(* Logix 5000 Controller export Example_PLC; controller Example_PLC 1769-L32E rev 19.11; software revision 19.01; part 3 of 6 *)

ADD_ON_INSTRUCTION AKD_Set_Parameter   (* revision 2.0, ExecutePrescan, ExecuteEnableInFalse *)
// Set Drive Parameter
VAR_OUTPUT
   DN : BOOL; {access Read Only, visible}   // Command Successful
   ER : BOOL; {access Read Only, visible}   // Error
END_VAR
VAR_IN_OUT
   Axis : AKD_Axis; {required}
END_VAR
VAR_INPUT
   Parameter_Number : INT; {visible}   // See help (F1) for parameter list.
   Parameter_Value : DINT; {required}   // Parameter Value
END_VAR
VAR
   Command_Timeout : TIMER := (PRE := 10000);   // Timeout Timer
   Command_Message_Type : SINT;   // Command Message Type
   Command_Axis_Number : SINT;   // Command Axis Number
   Step : SINT;
   Command_Bytes : SINT[8];
   OS_LoadStart : BOOL;
   Temp_Bytes : SINT[2];   // Temporary Bytes to Split into Command Bytes
END_VAR

ROUTINE EnableInFalse   (* ladder *)
// EnableIn_False
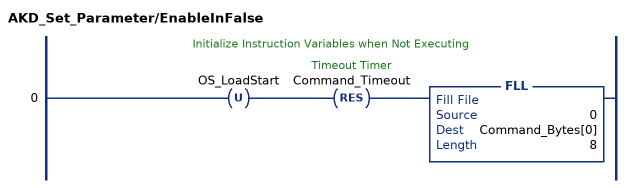
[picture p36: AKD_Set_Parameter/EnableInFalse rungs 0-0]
   // Initialize Instruction Variables when Not Executing
   0: OTU(OS_LoadStart)RES(Command_Timeout)FLL(0,Command_Bytes[0],8);
END_ROUTINE

ROUTINE Logic   (* ladder *)
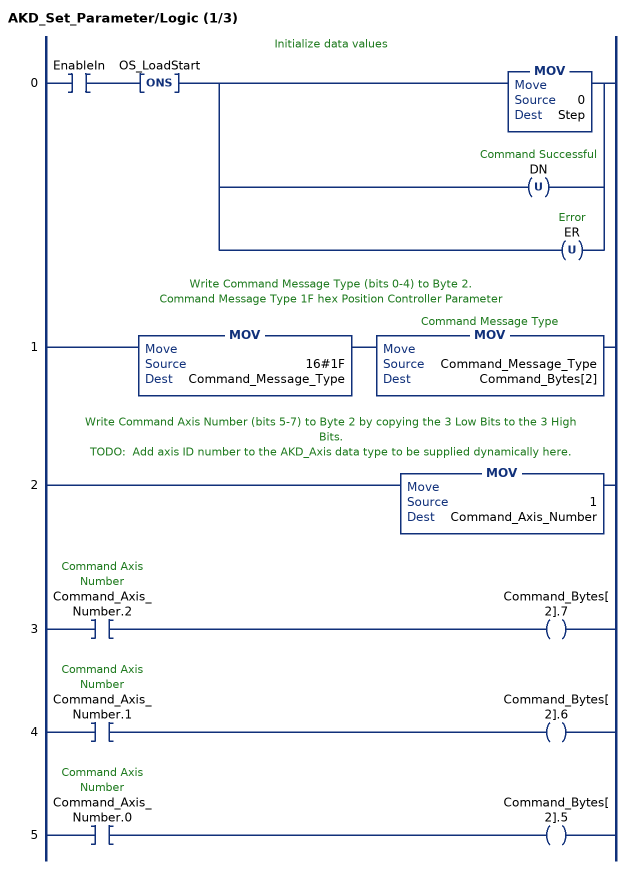
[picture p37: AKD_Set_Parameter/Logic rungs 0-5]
   // Initialize data values
   0: XIC(EnableIn)ONS(OS_LoadStart)[MOV(0,Step) ,OTU(DN) ,OTU(ER) ];
   // Write Command Message Type (bits 0-4) to Byte 2.
   // Command Message Type 1F hex Position Controller Parameter
   1: MOV(16#1F,Command_Message_Type)MOV(Command_Message_Type,Command_Bytes[2]);
   // Write Command Axis Number (bits 5-7) to Byte 2 by copying the 3 Low Bits to the 3 High Bits.
   // TODO:  Add axis ID number to the AKD_Axis data type to be supplied dynamically here.
   2: MOV(1,Command_Axis_Number);
   3: XIC(Command_Axis_Number.2)OTE(Command_Bytes[2].7);
   4: XIC(Command_Axis_Number.1)OTE(Command_Bytes[2].6);
   5: XIC(Command_Axis_Number.0)OTE(Command_Bytes[2].5);
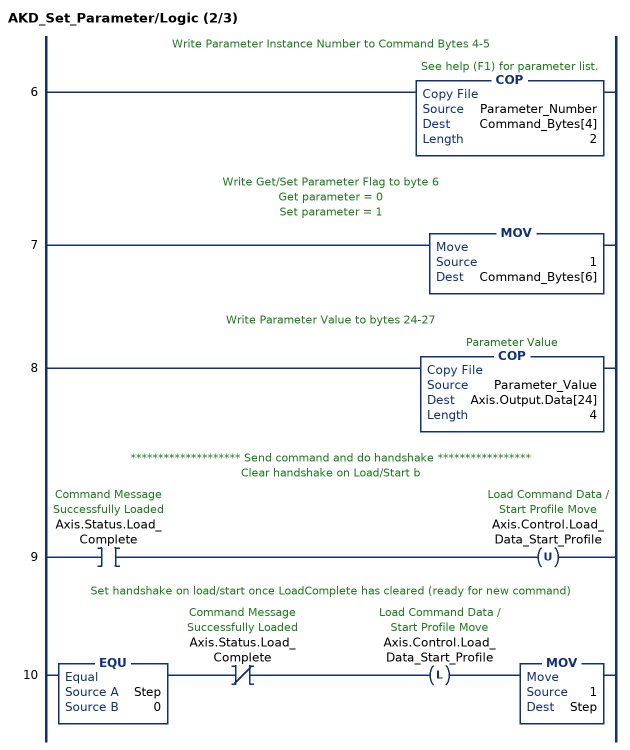
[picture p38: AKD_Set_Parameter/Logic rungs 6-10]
   // Write Parameter Instance Number to Command Bytes 4-5
   6: COP(Parameter_Number,Command_Bytes[4],2);
   // Write Get/Set Parameter Flag to byte 6
   // Get parameter = 0
   // Set parameter = 1
   7: MOV(1,Command_Bytes[6]);
   // Write Parameter Value to bytes 24-27
   8: COP(Parameter_Value,Axis.Output.Data[24],4);
   // ******************** Send command and do handshake *****************
   // Clear handshake on Load/Start b
   9: XIC(Axis.Status.Load_Complete)OTU(Axis.Control.Load_Data_Start_Profile);
   // Set handshake on load/start once LoadComplete has cleared (ready for new command)
   10: EQU(Step,0)XIO(Axis.Status.Load_Complete)OTL(Axis.Control.Load_Data_Start_Profile)MOV(1,Step);
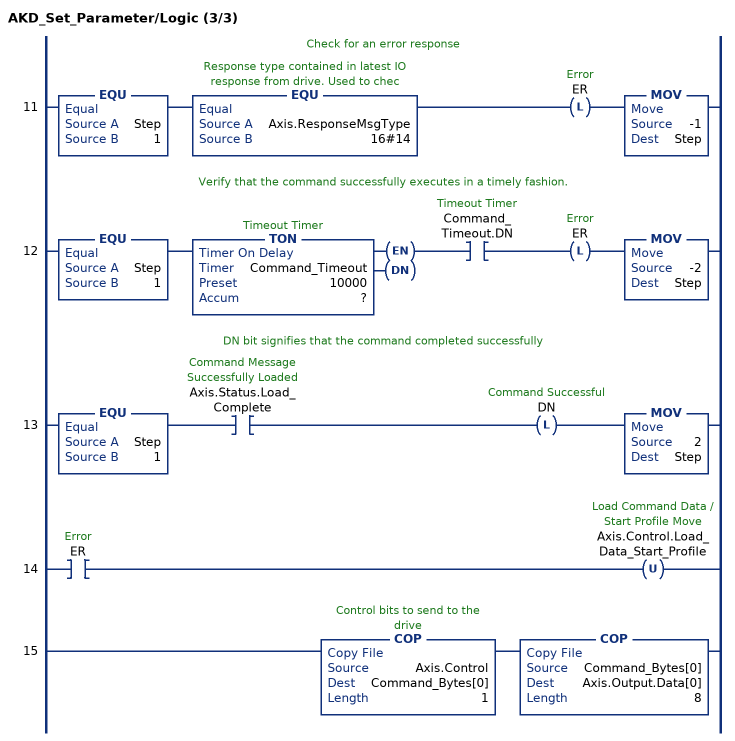
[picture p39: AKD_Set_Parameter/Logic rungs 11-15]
   // Check for an error response
   11: EQU(Step,1)EQU(Axis.ResponseMsgType,16#14)OTL(ER)MOV(-1,Step);
   // Verify that the command successfully executes in a timely fashion.
   12: EQU(Step,1)TON(Command_Timeout,?,?)XIC(Command_Timeout.DN)OTL(ER)MOV(-2,Step);
   // DN bit signifies that the command completed successfully
   13: EQU(Step,1)XIC(Axis.Status.Load_Complete)OTL(DN)MOV(2,Step);
   14: XIC(ER)OTU(Axis.Control.Load_Data_Start_Profile);
   15: COP(Axis.Control,Command_Bytes[0],1)COP(Command_Bytes[0],Axis.Output.Data[0],8);
END_ROUTINE

ROUTINE Prescan   (* ladder *)
// Prescan
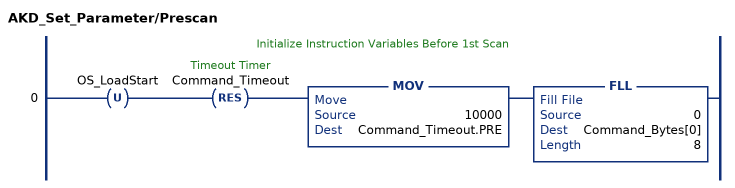
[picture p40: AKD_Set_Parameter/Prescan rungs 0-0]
   // Initialize Instruction Variables Before 1st Scan
   0: OTU(OS_LoadStart)RES(Command_Timeout)MOV(10000,Command_Timeout.PRE)FLL(0,Command_Bytes[0],8);
END_ROUTINE
END_ADD_ON_INSTRUCTION

ADD_ON_INSTRUCTION AKD_Fault_Reset_RevB   (* revision 3.0, ExecutePrescan, ExecuteEnableInFalse *)
// Drive Fault Reset
VAR_OUTPUT
   DN : BOOL; {access Read Only, visible}   // Command Successful
   ER : BOOL; {access Read Only, visible}   // Error
END_VAR
VAR_IN_OUT
   Axis : AKD_Axis; {required}
END_VAR
VAR
   Step : SINT;
   Set_Parameter : AKD_Set_Parameter := (Parameter_Number := 113);
END_VAR

ROUTINE EnableInFalse   (* ladder *)
// EnableIn_False
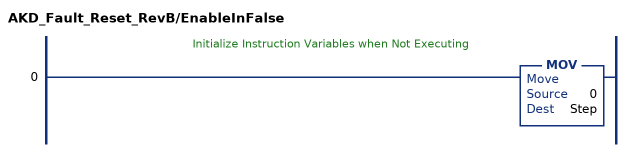
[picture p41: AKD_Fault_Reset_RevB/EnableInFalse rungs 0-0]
   // Initialize Instruction Variables when Not Executing
   0: MOV(0,Step);
END_ROUTINE

ROUTINE Logic   (* ladder *)
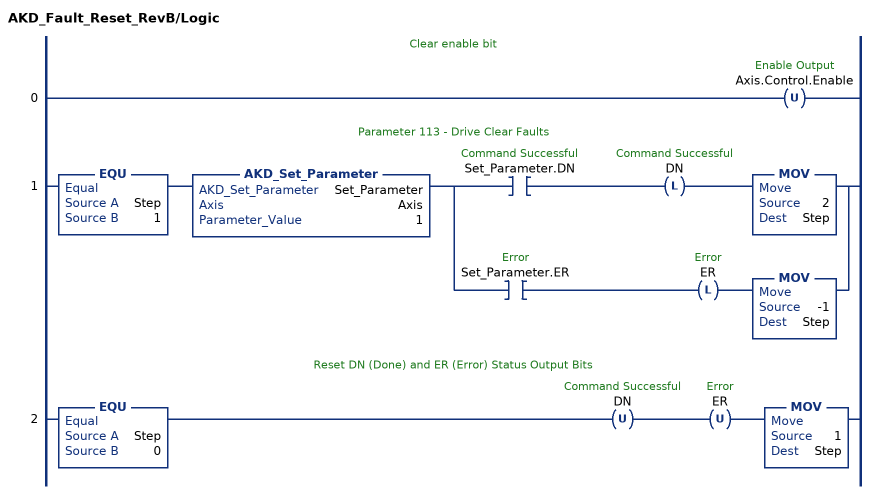
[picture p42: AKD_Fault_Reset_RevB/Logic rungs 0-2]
   // Clear enable bit
   0: OTU(Axis.Control.Enable);
   // Parameter 113 - Drive Clear Faults
   1: EQU(Step,1)AKD_Set_Parameter(Set_Parameter,Axis,1)[XIC(Set_Parameter.DN) OTL(DN) MOV(2,Step) ,XIC(Set_Parameter.ER) OTL(ER) MOV(-1,Step) ];
   // Reset DN (Done) and ER (Error) Status Output Bits
   2: EQU(Step,0)OTU(DN)OTU(ER)MOV(1,Step);
END_ROUTINE

ROUTINE Prescan   (* ladder *)
// Prescan
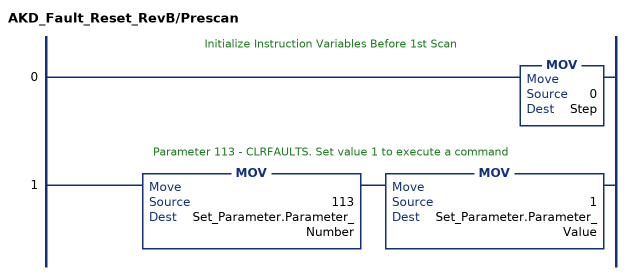
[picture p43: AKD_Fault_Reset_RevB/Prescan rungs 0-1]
   // Initialize Instruction Variables Before 1st Scan
   0: MOV(0,Step);
   // Parameter 113 - CLRFAULTS. Set value 1 to execute a command
   1: MOV(113,Set_Parameter.Parameter_Number)MOV(1,Set_Parameter.Parameter_Value);
END_ROUTINE
END_ADD_ON_INSTRUCTION

ADD_ON_INSTRUCTION AKD_Get_Attribute   (* revision 2.1, ExecutePrescan, ExecuteEnableInFalse *)
// Get Position Controller Attribute
// Revision note:
// Don't error if Command_Timeout preset is 0
VAR_OUTPUT
   DN : BOOL; {access Read Only, visible}   // Command Successful
   ER : BOOL; {access Read Only, visible}   // Error
END_VAR
VAR_IN_OUT
   Axis : AKD_Axis; {required}
END_VAR
VAR_INPUT
   Attribute_Number : INT; {visible}   // Attribute Number (see help for options)
END_VAR
VAR_OUTPUT
   Attribute_Value : DINT; {access Read Only, required}   // Attribute Value
END_VAR
VAR
   Command_Timeout : TIMER := (PRE := 100);   // Timeout Timer
   OS_LoadStart : BOOL;
   ErrorSource : SINT;
END_VAR

ROUTINE EnableInFalse   (* ladder *)
// EnableIn_False
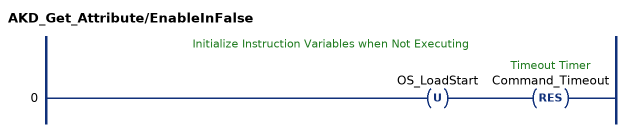
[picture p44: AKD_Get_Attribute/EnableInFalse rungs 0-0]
   // Initialize Instruction Variables when Not Executing
   0: OTU(OS_LoadStart)RES(Command_Timeout);
END_ROUTINE

ROUTINE Logic   (* ladder *)
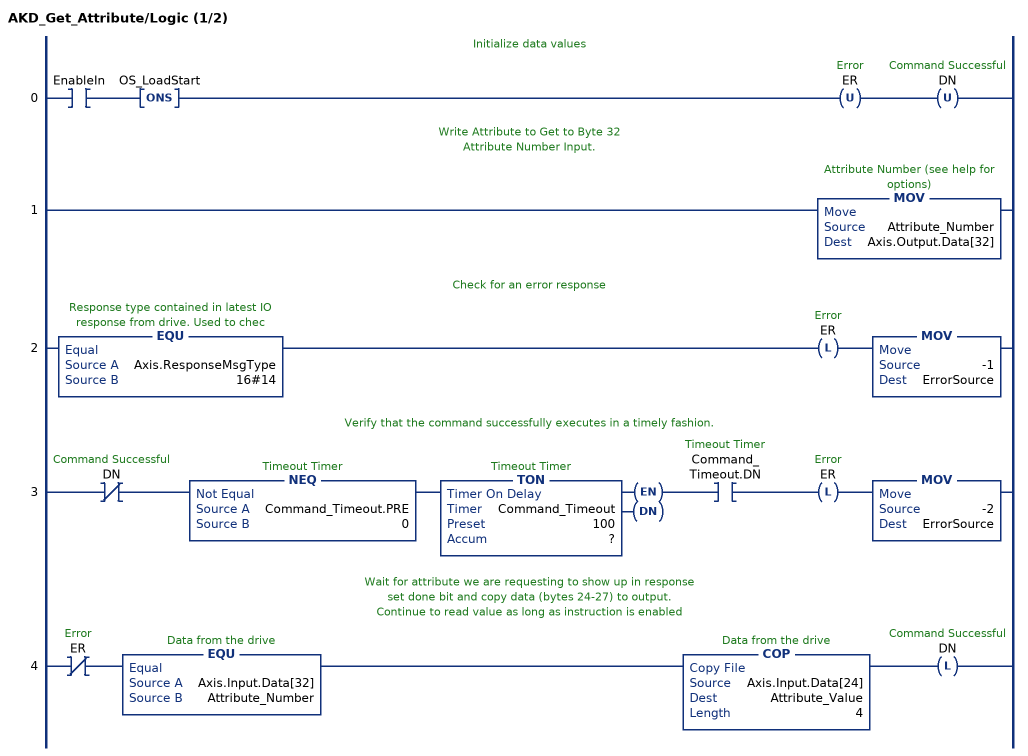
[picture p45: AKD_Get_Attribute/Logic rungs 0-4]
   // Initialize data values
   0: XIC(EnableIn)ONS(OS_LoadStart)OTU(ER)OTU(DN);
   // Write Attribute to Get to Byte 32
   // Attribute Number Input.
   1: MOV(Attribute_Number,Axis.Output.Data[32]);
   // Check for an error response
   2: EQU(Axis.ResponseMsgType,16#14)OTL(ER)MOV(-1,ErrorSource);
   // Verify that the command successfully executes in a timely fashion.
   3: XIO(DN)NEQ(Command_Timeout.PRE,0)TON(Command_Timeout,?,?)XIC(Command_Timeout.DN)OTL(ER)MOV(-2,ErrorSource);
   // Wait for attribute we are requesting to show up in response
   // set done bit and copy data (bytes 24-27) to output.
   // Continue to read value as long as instruction is enabled
   4: XIO(ER)EQU(Axis.Input.Data[32],Attribute_Number)COP(Axis.Input.Data[24],Attribute_Value,4)OTL(DN);
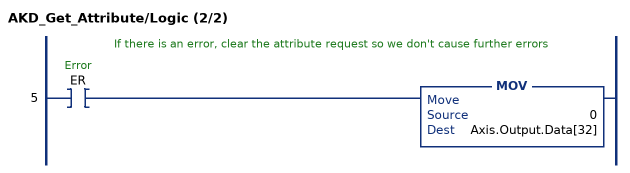
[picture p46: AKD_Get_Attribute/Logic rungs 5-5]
   // If there is an error, clear the attribute request so we don't cause further errors
   5: XIC(ER)MOV(0,Axis.Output.Data[32]);
END_ROUTINE

ROUTINE Prescan   (* ladder *)
// Prescan
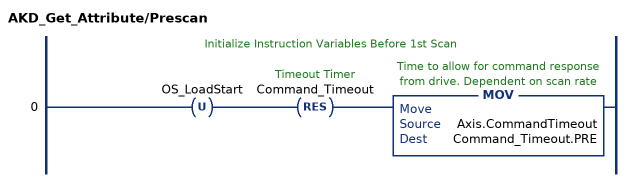
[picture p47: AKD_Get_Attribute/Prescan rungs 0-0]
   // Initialize Instruction Variables Before 1st Scan
   0: OTU(OS_LoadStart)RES(Command_Timeout)MOV(Axis.CommandTimeout,Command_Timeout.PRE);
END_ROUTINE
END_ADD_ON_INSTRUCTION

ADD_ON_INSTRUCTION AKD_Set_Attribute   (* revision 2.1, ExecutePrescan, ExecuteEnableInFalse *)
// Set Position Controller Attribute
// Revision note:
// Don't error if Command_Timeout preset is 0
VAR_OUTPUT
   DN : BOOL; {access Read Only, visible}   // Command Successful
   ER : BOOL; {access Read Only, visible}   // Error
END_VAR
VAR_IN_OUT
   Axis : AKD_Axis; {required}
END_VAR
VAR_INPUT
   Attribute_Number : INT; {visible}   // Attribute Number (see help for options)
   Attribute_Value : DINT; {required}   // Attribute Value
END_VAR
VAR
   Command_Timeout : TIMER := (PRE := 200);   // Timeout Timer
   Command_Message_Type : SINT;   // Command Message Type
   Command_Axis_Number : SINT;   // Command Axis Number
   Step : SINT;
   Command_Bytes : SINT[8];
   OS_LoadStart : BOOL;
END_VAR

ROUTINE EnableInFalse   (* ladder *)
// EnableIn_False
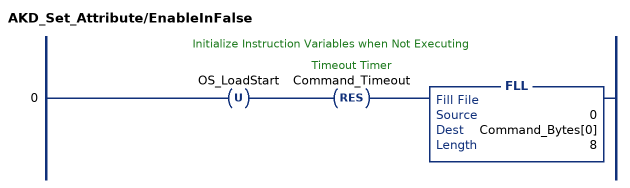
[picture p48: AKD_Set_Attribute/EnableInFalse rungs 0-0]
   // Initialize Instruction Variables when Not Executing
   0: OTU(OS_LoadStart)RES(Command_Timeout)FLL(0,Command_Bytes[0],8);
END_ROUTINE

ROUTINE Logic   (* ladder *)
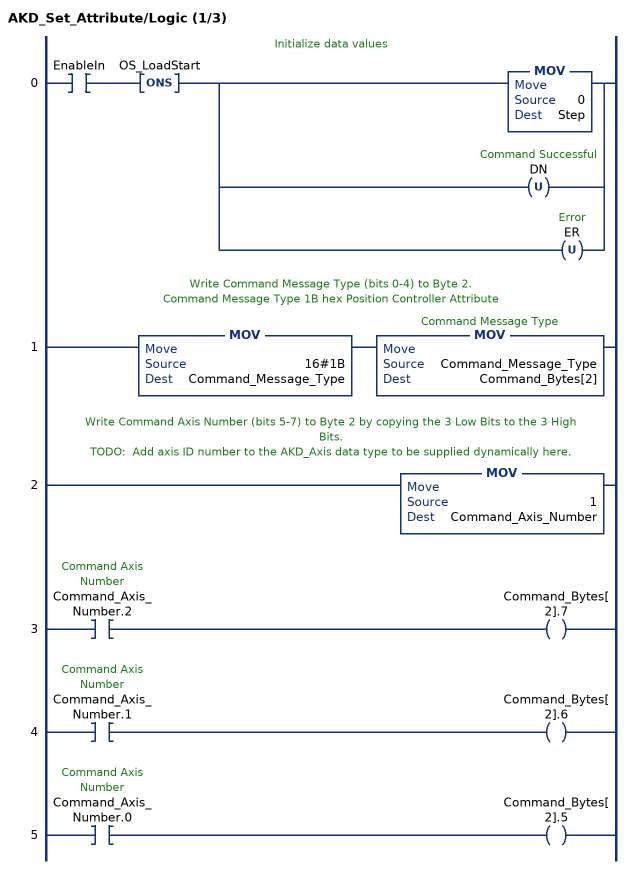
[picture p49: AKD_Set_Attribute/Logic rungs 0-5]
   // Initialize data values
   0: XIC(EnableIn)ONS(OS_LoadStart)[MOV(0,Step) ,OTU(DN) ,OTU(ER) ];
   // Write Command Message Type (bits 0-4) to Byte 2.
   // Command Message Type 1B hex Position Controller Attribute
   1: MOV(16#1B,Command_Message_Type)MOV(Command_Message_Type,Command_Bytes[2]);
   // Write Command Axis Number (bits 5-7) to Byte 2 by copying the 3 Low Bits to the 3 High Bits.
   // TODO:  Add axis ID number to the AKD_Axis data type to be supplied dynamically here.
   2: MOV(1,Command_Axis_Number);
   3: XIC(Command_Axis_Number.2)OTE(Command_Bytes[2].7);
   4: XIC(Command_Axis_Number.1)OTE(Command_Bytes[2].6);
   5: XIC(Command_Axis_Number.0)OTE(Command_Bytes[2].5);
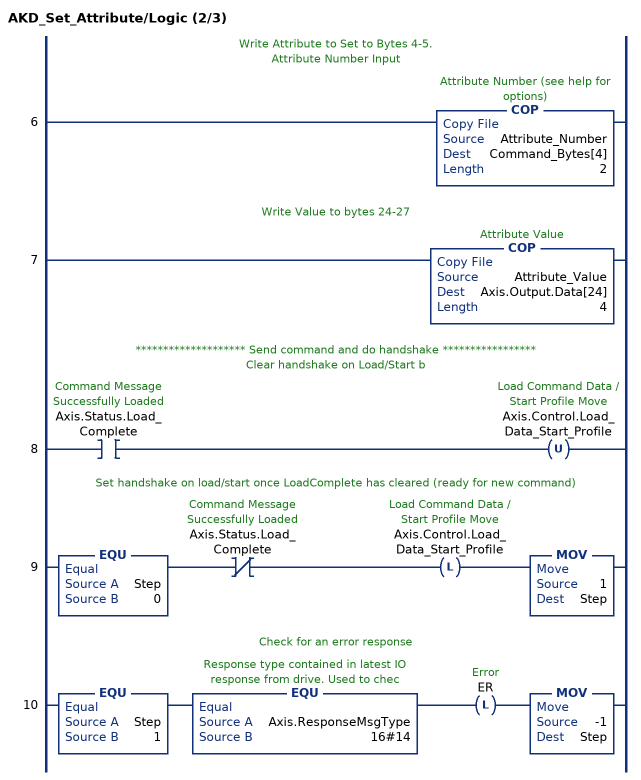
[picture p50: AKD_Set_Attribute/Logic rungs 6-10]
   // Write Attribute to Set to Bytes 4-5.
   // Attribute Number Input
   6: COP(Attribute_Number,Command_Bytes[4],2);
   // Write Value to bytes 24-27
   7: COP(Attribute_Value,Axis.Output.Data[24],4);
   // ******************** Send command and do handshake *****************
   // Clear handshake on Load/Start b
   8: XIC(Axis.Status.Load_Complete)OTU(Axis.Control.Load_Data_Start_Profile);
   // Set handshake on load/start once LoadComplete has cleared (ready for new command)
   9: EQU(Step,0)XIO(Axis.Status.Load_Complete)OTL(Axis.Control.Load_Data_Start_Profile)MOV(1,Step);
   // Check for an error response
   10: EQU(Step,1)EQU(Axis.ResponseMsgType,16#14)OTL(ER)MOV(-1,Step);
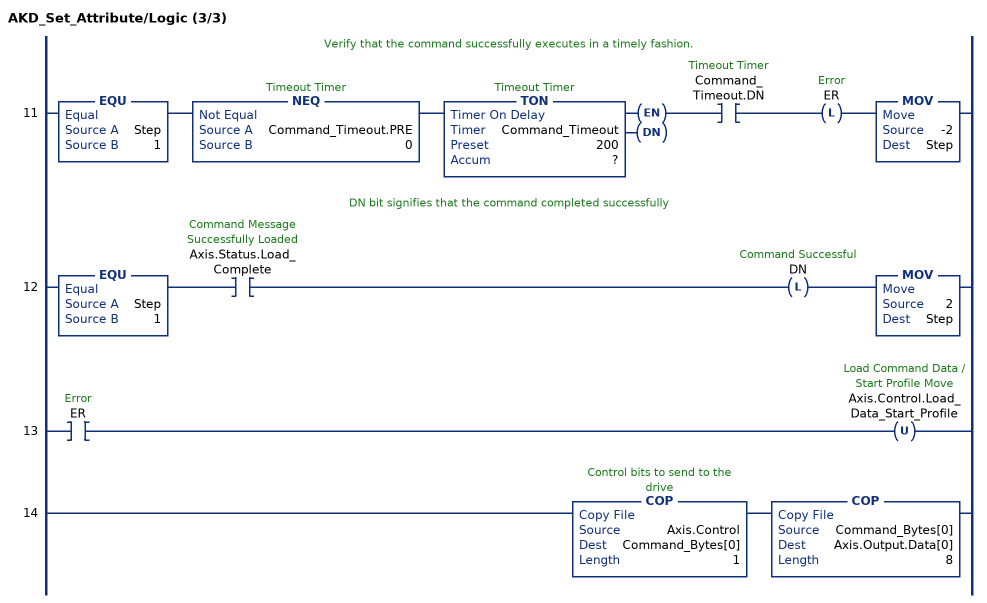
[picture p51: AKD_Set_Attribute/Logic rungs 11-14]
   // Verify that the command successfully executes in a timely fashion.
   11: EQU(Step,1)NEQ(Command_Timeout.PRE,0)TON(Command_Timeout,?,?)XIC(Command_Timeout.DN)OTL(ER)MOV(-2,Step);
   // DN bit signifies that the command completed successfully
   12: EQU(Step,1)XIC(Axis.Status.Load_Complete)OTL(DN)MOV(2,Step);
   13: XIC(ER)OTU(Axis.Control.Load_Data_Start_Profile);
   14: COP(Axis.Control,Command_Bytes[0],1)COP(Command_Bytes[0],Axis.Output.Data[0],8);
END_ROUTINE

ROUTINE Prescan   (* ladder *)
// Prescan
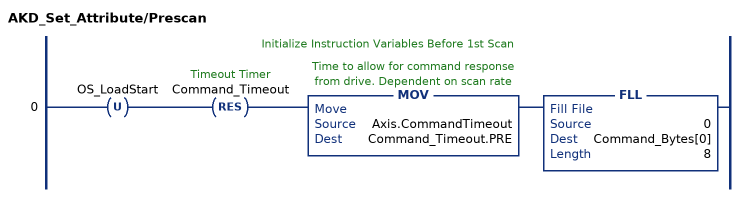
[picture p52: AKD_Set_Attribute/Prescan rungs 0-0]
   // Initialize Instruction Variables Before 1st Scan
   0: OTU(OS_LoadStart)RES(Command_Timeout)MOV(Axis.CommandTimeout,Command_Timeout.PRE)FLL(0,Command_Bytes[0],8);
END_ROUTINE
END_ADD_ON_INSTRUCTION

ADD_ON_INSTRUCTION AKD_Set_Mode   (* revision 2.2, ExecutePrescan, ExecuteEnableInFalse *)
// Set Drive Mode
// Revision note:
// Recover properly from errors (previously could not recover if AKD_Set_Attribute errored)
VAR_IN_OUT
   Axis : AKD_Axis; {required}
END_VAR
VAR_INPUT
   Mode_Requested : SINT; {required}   // Drive Mode Requested (0=Position, 1=Velocity, 2=Torque)
END_VAR
VAR_OUTPUT
   DN : BOOL; {access Read Only, visible}   // Command Successfully Initiated
   ER : BOOL; {access Read Only, visible}   // Error
   Mode_Actual : SINT; {access Read Only, required}   // Drive Mode Actual (0=Position, 1=Velocity, 2=Torque)
END_VAR
VAR
   Accel_Internal : DINT;   // Scaled Accel Value for Drive
   Step : SINT;   // Sequence Step Number
   ErrorSource : SINT;   // Source of Error
   StartONS : BOOL;
   Pause_Timer : TIMER;   // Pause During Jog Command Sequence
   Get_Mode : AKD_Get_Attribute := (Attribute_Number := 3);
   Set_Mode : AKD_Set_Attribute := (Attribute_Number := 3);
   Command_Timeout : TIMER := (PRE := 100);
END_VAR

ROUTINE EnableInFalse   (* ladder *)
// EnableIn_False
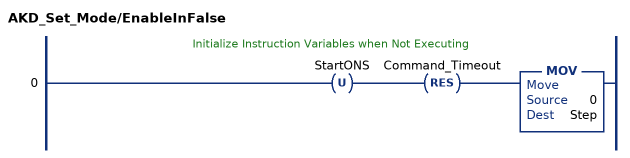
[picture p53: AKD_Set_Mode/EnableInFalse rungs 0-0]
   // Initialize Instruction Variables when Not Executing
   0: OTU(StartONS)RES(Command_Timeout)MOV(0,Step);
END_ROUTINE
